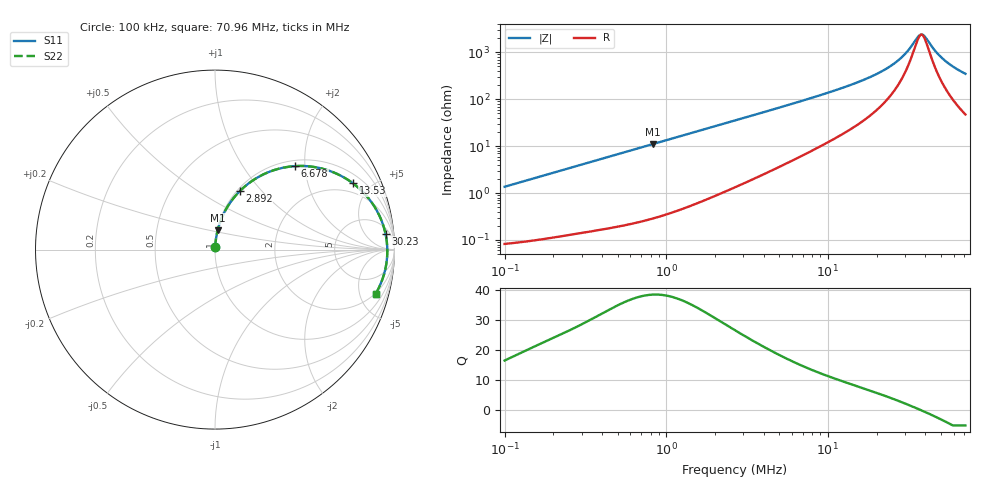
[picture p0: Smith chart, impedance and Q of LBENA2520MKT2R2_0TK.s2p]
! LBENA2520MKT2R2_0TK  S-PARAMETER MODEL  ( Standard Model )
! Model Generated by TAIYO YUDEN Corporation (http://www.ty-top.com)
! Version 1.0
! TAIYO YUDEN Control No. 20240828
! Copyright(c) 2024 TAIYO YUDEN CO.,LTD. All Rights Reserved.
! Product Description (link to TY-COMPAS)
! https://ds.yuden.co.jp/TYCOMPAS/or/detail?pn=LBENA2520MKT2R2M0TK&u=M
! Products Name : Inductors
! Characteristics :
!  Inductance : 2.2 [uH] , SRF(min) : - [Hz] , DC Resistance(max) : 0.077 [Ohm]
!  Rated Current : Saturation  3000 [mA] , Temp Rise  2400 [mA] (40 [degC])
!  Case Size : 2.5 x 2.0 / 0.098 x 0.079 [mm/inch] , Thickness : 1.2 / 0.047 [mm/inch]
!  (Conditions: Temperature = 25 [degC] , DC Bias Current = 0 [A])
! External Node Assignments :
!  1  o---GGG---o  2
! GND o---------o GND
! Frequency Range : 0.1MHz  -  70.9631MHz  [ 402 STEP ]
# MHz S RI R 50
! Freq[MHz].  S11 Real  S11 Imag  S21 Real  S21 Imag  S12 Real  S12 Imag  S22 Real  S22 Imag
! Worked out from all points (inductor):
!   401 points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, 100 kHz to 70.96 MHz, reference 50 ohm
!   read as one part in series: L = 2.16 uH near 103.3 kHz
!   highest Q = 38.3 at 830.7 kHz (marker M1), where L = 2.12 uH
!   self-resonance near 37.92 MHz
!   S11 on the Smith chart (normalised r, x): 100 kHz: 1.00, +0.03; 2.892 MHz: 1.03, +0.76; 6.678 MHz: 1.12, +1.78; 13.53 MHz: 1.44, +3.90; 30.23 MHz: 9, +17; 70.96 MHz: 1.95, -6.92
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0.1  0.00101 0.0136  0.999 -0.0136  0.999 -0.0136  0.00101 0.0136
0.300295  0.00303 0.0401  0.997 -0.0401  0.997 -0.0401  0.00303 0.0401
0.830726  0.0148 0.1085  0.9852 -0.1085  0.9852 -0.1085  0.0148 0.1085
0.90177  0.0171 0.1174  0.9829 -0.1174  0.9829 -0.1174  0.0171 0.1174
1.682457  0.0531 0.2095  0.9469 -0.2095  0.9469 -0.2095  0.0531 0.2095
2.70797  0.1226 0.3095  0.8774 -0.3095  0.8774 -0.3095  0.1226 0.3095
2.891706  0.1369 0.3246  0.8631 -0.3246  0.8631 -0.3246  0.1369 0.3246
4.287619  0.2536 0.4111  0.7464 -0.4111  0.7464 -0.4111  0.2536 0.4111
6.678222  0.4463 0.4652  0.5537 -0.4652  0.5537 -0.4652  0.4463 0.4652
7.999526  0.5348 0.4627  0.4652 -0.4627  0.4652 -0.4627  0.5348 0.4627
13.5253  0.7692 0.3689  0.2308 -0.3689  0.2308 -0.3689  0.7692 0.3689
18.78013  0.8719 0.2643  0.1281 -0.2643  0.1281 -0.2643  0.8719 0.2643
24.02217  0.9224 0.175  0.0776 -0.175  0.0776 -0.175  0.9224 0.175
27.39258  0.9404 0.1255  0.0596 -0.1255  0.0596 -0.1255  0.9404 0.1255
30.22723  0.9501 0.0878  0.0499 -0.0878  0.0499 -0.0878  0.9501 0.0878
36.20777  0.9594 0.018  0.0406 -0.018  0.0406 -0.018  0.9594 0.018
38.66447  0.9601 -0.00756  0.0399 0.00756  0.0399 0.00756  0.9601 -0.00756
40.61578  0.9597 -0.0268  0.0403 0.0268  0.0403 0.0268  0.9597 -0.0268
47.08071  0.9538 -0.0847  0.0462 0.0847  0.0462 0.0847  0.9538 -0.0847
51.95275  0.9456 -0.1234  0.0544 0.1234  0.0544 0.1234  0.9456 -0.1234
60.22222  0.9267 -0.1813  0.0733 0.1813  0.0733 0.1813  0.9267 -0.1813
70.9631  0.8958 -0.2447  0.1042 0.2447  0.1042 0.2447  0.8958 -0.2447
